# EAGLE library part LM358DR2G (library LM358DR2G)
LM358DR2G, Dual Operational Amplifier 5 to 28V, 8-Pin SOIC Source: Datasheet
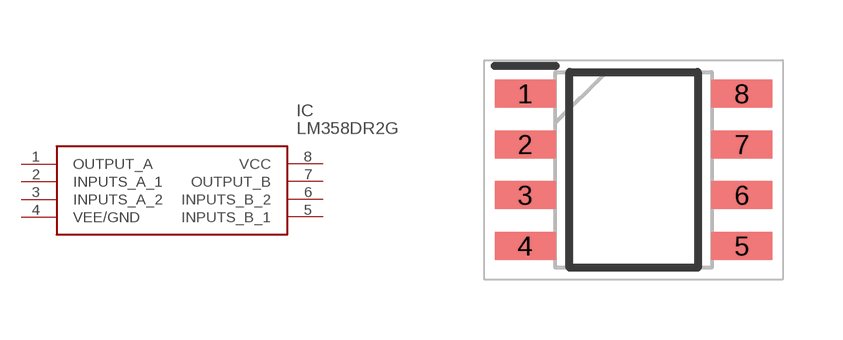
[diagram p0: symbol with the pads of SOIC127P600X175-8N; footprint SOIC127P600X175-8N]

Designator prefix IC

## LM358DR2G (Arrow_Part_Number: LM358DR2G; Arrow_Price-Stock: null?region=asia; Description: LM358DR2G, Dual Operational Amplifier 5 to 28V, 8-Pin SOIC; Height: 1.75mm; Manufacturer_Name: onsemi; Manufacturer_Part_Number: LM358DR2G; Mouser_Part_Number: 863-LM358DR2G; Mouser_Price-Stock: https://www.mouser.co.uk/ProductDetail/onsemi/LM358DR2G?qs=2OtswVQKCOFTvDtJvQ3XHw%3D%3D)  [SOIC127P600X175-8N]
1  OUTPUT_A
2  INPUTS_A_1
3  INPUTS_A_2
4  VEE/GND
5  INPUTS_B_1
6  INPUTS_B_2
7  OUTPUT_B
8  VCC

## Footprint SOIC127P600X175-8N (pad centres in mm)
SOIC 8, 150 mils
smd 1.525 x 0.7: 1 -2.712,1.905; 2 -2.712,0.635; 3 -2.712,-0.635; 4 -2.712,-1.905; 5 2.712,-1.905; 6 2.712,-0.635; 7 2.712,0.635; 8 2.712,1.905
